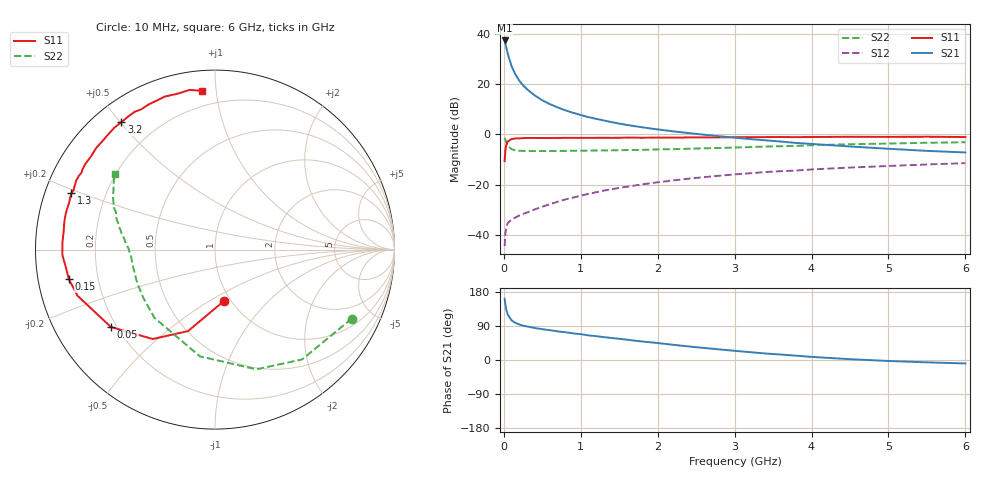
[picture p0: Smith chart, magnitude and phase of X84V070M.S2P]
! SIEMENS Small Signal Semiconductors
! BFP136W
! Si NPN RF Bipolar Junction Transistor in SOT343
! VCE = 4 V  IC = 70 mA
! Common Emitter S-Parameters:  September  1994
# GHz  S  MA  R  50
!  f  S11  S21  S12  S22
! GHz  MAG  ANG  MAG  ANG  MAG  ANG  MAG  ANG
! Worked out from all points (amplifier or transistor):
!   40 points, 10 MHz to 6 GHz, reference 50 ohm
!   highest |S21| = 37.5 dB at 10 MHz (marker M1)
!   |S21| within 3 dB of that: start of sweep to 33.84 MHz
!   unconditionally stable (mu >= 1): 578.3 MHz to 2.886 GHz
!   at 200 MHz: K = 0.61, MSG = 26.9 dB, |S12| = -32.4 dB
!   at 1.5 GHz: K = 1.10, MAG = 10.9 dB, |S12| = -21.3 dB
!   at 6 GHz: K = 0.96, MSG = 2.1 dB, |S12| = -11.4 dB
!   S11 on the Smith chart (normalised r, x): 10 MHz: 0.92, -0.58; 50 MHz: 0.18, -0.32; 150 MHz: 0.09, -0.10; 1.3 GHz: 0.08, +0.19; 3.2 GHz: 0.08, +0.50; 6 GHz: 0.11, +0.92
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0.01  0.2921 -80.6  75.03 161.7  0.0059 72.9  0.853 -26.8
0.02  0.478 -108.3  65.6 146.2  0.0105 58.8  0.7811 -51.6
0.03  0.6066 -124.8  56.47 134.7  0.0136 51.0  0.7058 -70.9
0.05  0.7226 -143.3  41.09 120.2  0.0171 39.4  0.6009 -98.0
0.1  0.8084 -161.5  23.08 104.8  0.0199 33.9  0.5083 -131.6
0.15  0.8314 -168.7  15.75 97.9  0.022 34.9  0.4811 -146.3
0.2  0.8357 -172.8  11.86 93.8  0.0241 37.9  0.4724 -154.4
0.25  0.8445 -176.0  9.565 90.8  0.0259 40.3  0.4691 -159.5
0.3  0.8511 -178.1  8.004 88.5  0.0277 43.0  0.4667 -163.0
0.4  0.8511 177.8  6.032 84.5  0.0319 47.3  0.4659 -167.6
0.5  0.8495 175.1  4.809 81.3  0.0361 51.0  0.4661 -170.7
0.6  0.8493 172.9  4.013 78.6  0.0407 53.2  0.4675 -172.6
0.7  0.8526 170.4  3.456 75.5  0.0455 55.5  0.4687 -174.1
0.9  0.855 166.8  2.705 70.4  0.0549 57.4  0.471 -176.7
1.1  0.8536 162.4  2.212 65.0  0.0653 58.7  0.4754 -178.2
1.3  0.8597 158.6  1.901 60.3  0.0758 59.1  0.4801 -179.9
1.7  0.8627 151.6  1.464 51.0  0.0957 57.7  0.4906 177.1
2.2  0.8639 143.3  1.153 40.2  0.1208 54.7  0.5082 173.5
3.2  0.881 126.3  0.808 20.7  0.1681 45.9  0.559 164.8
4.5  0.8974 108.2  0.575 2.2  0.2184 33.9  0.6381 152.9
5.5  0.9009 99.0  0.47 -6.2  0.2518 26.1  0.682 145.8
6  0.8874 94.7  0.437 -9.1  0.268 21.7  0.6988 142.8
